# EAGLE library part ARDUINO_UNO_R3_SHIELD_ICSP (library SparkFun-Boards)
Arduino R3 Shield Footprint with ICSP Header Includes pins for 6-pin (2x3) ICSP Header. Compatible with Leonardo boards that require SPI pin connections via this header. SparkFun Products: CryptoShield microSD Shield R3 Stackable Headers Kit
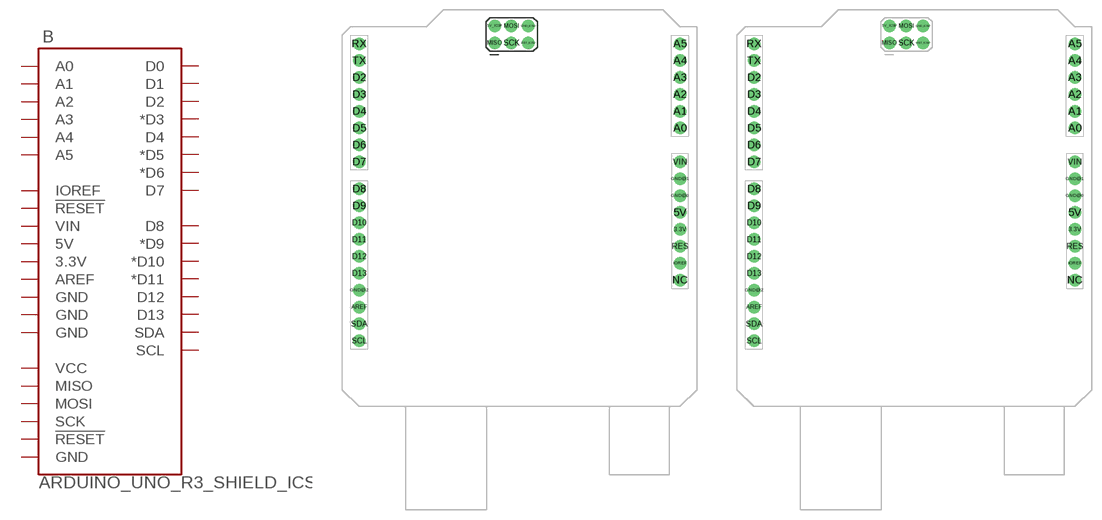
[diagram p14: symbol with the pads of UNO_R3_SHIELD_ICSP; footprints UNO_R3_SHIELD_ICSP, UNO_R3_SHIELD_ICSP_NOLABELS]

Designator prefix B

## ARDUINO_UNO_R3_SHIELD_ICSP  [UNO_R3_SHIELD_ICSP]
3.3V  3.3V
5V  5V
5V_ICSP  VCC
A0  A0
A1  A1
A2  A2
A3  A3
A4  A4
A5  A5
AREF  AREF
D2  D2
D3  *D3
D4  D4
D5  *D5
D6  *D6
D7  D7
D8  D8
D9  *D9
D10  *D10
D11  *D11
D12  D12
D13  D13
GND@0  GND
GND@1  GND
GND@2  GND
GND_ICSP  GND
IOREF  IOREF
MISO  MISO
MOSI  MOSI
RES  !RESET!
RST_ICSP  !RESET!
RX  D0
SCK  SCK
SCL  SCL
SDA  SDA
TX  D1
VIN  VIN

## ARDUINO_UNO_R3_SHIELD_ICSP-NO_LABELS  [UNO_R3_SHIELD_ICSP_NOLABELS]
Pads as for UNO_R3_SHIELD_ICSP

## Footprint UNO_R3_SHIELD_ICSP (pad centres in mm)
Arduino Uno-Compatible Footprint with ICSP No mounting holes. Specifications: Pin count: 38 Pin pitch: 0.1" Area:2.1x2.35" Example device(s): Arduino Uno R3 Shield ICSP
drill 1.016 pad 1.88: 3.3V 24.13,-3.81; 5V 24.13,-1.27; 5V_ICSP -3.76,26.81; A0 24.13,11.43; A1 24.13,13.97; A2 24.13,16.51; A3 24.13,19.05; A4 24.13,21.59; A5 24.13,24.13; AREF -24.13,-15.494; D2 -24.13,19.05; D3 -24.13,16.51; D4 -24.13,13.97; D5 -24.13,11.43; D6 -24.13,8.89; D7 -24.13,6.35; D8 -24.13,2.286; D9 -24.13,-0.254; D10 -24.13,-2.794; D11 -24.13,-5.334; D12 -24.13,-7.874; D13 -24.13,-10.414; GND@0 24.13,1.27; GND@1 24.13,3.81; GND@2 -24.13,-12.954; GND_ICSP 1.32,26.81; IOREF 24.13,-8.89; MISO -3.76,24.27; MOSI -1.22,26.81; NC 24.13,-11.43; RES 24.13,-6.35; RST_ICSP 1.32,24.27; RX -24.13,24.13; SCK -1.22,24.27; SCL -24.13,-20.574; SDA -24.13,-18.034; TX -24.13,21.59; VIN 24.13,6.35

## Footprint UNO_R3_SHIELD_ICSP_NOLABELS (pad centres in mm)
Arduino Uno-Compatible Footprint with ICSP No mounting holes, no silk labels on pins. Specifications: Pin count: 38 Pin pitch: 0.1" Area:2.1x2.35" Example device(s): Arduino Uno R3 Shield ICSP
drill 1.016 pad 1.88: 3.3V 24.13,-3.81; 5V 24.13,-1.27; 5V_ICSP -3.76,26.81; A0 24.13,11.43; A1 24.13,13.97; A2 24.13,16.51; A3 24.13,19.05; A4 24.13,21.59; A5 24.13,24.13; AREF -24.13,-15.494; D2 -24.13,19.05; D3 -24.13,16.51; D4 -24.13,13.97; D5 -24.13,11.43; D6 -24.13,8.89; D7 -24.13,6.35; D8 -24.13,2.286; D9 -24.13,-0.254; D10 -24.13,-2.794; D11 -24.13,-5.334; D12 -24.13,-7.874; D13 -24.13,-10.414; GND@0 24.13,1.27; GND@1 24.13,3.81; GND@2 -24.13,-12.954; GND_ICSP 1.32,26.81; IOREF 24.13,-8.89; MISO -3.76,24.27; MOSI -1.22,26.81; NC 24.13,-11.43; RES 24.13,-6.35; RST_ICSP 1.32,24.27; RX -24.13,24.13; SCK -1.22,24.27; SCL -24.13,-20.574; SDA -24.13,-18.034; TX -24.13,21.59; VIN 24.13,6.35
